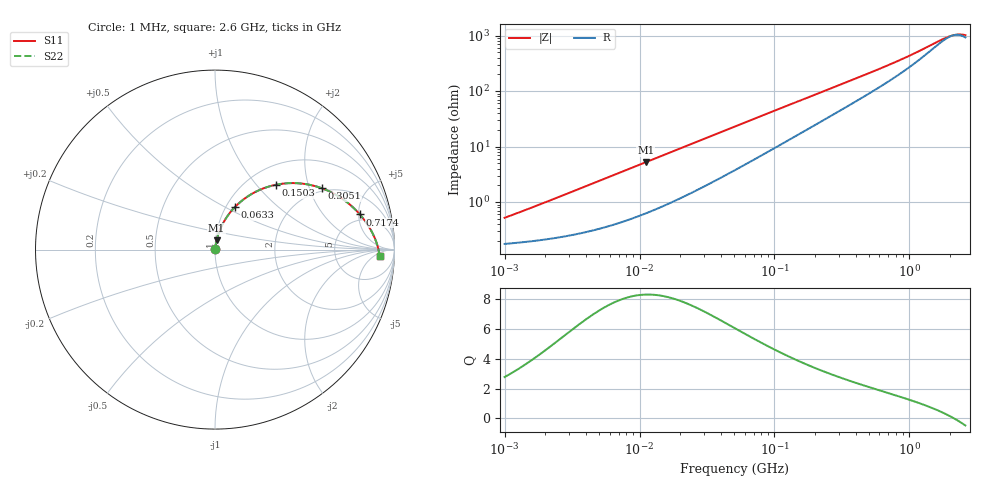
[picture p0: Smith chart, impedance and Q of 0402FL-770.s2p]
# MHz S MA R 50
!Freq  MagS11  AngS11  MagS21  AngS21  MagS12  AngS12  MagS22  AngS22
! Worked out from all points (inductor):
!   801 points, 1 MHz to 2.6 GHz, reference 50 ohm
!   read as one part in series: L = 77.1 nH near 1.103 MHz
!   highest Q = 8.32 at 11.11 MHz (marker M1), where L = 74 nH
!   self-resonance near 2.15 GHz
!   S11 on the Smith chart (normalised r, x): 1 MHz: 1.00, +0.01; 63.3 MHz: 1.10, +0.56; 150.3 MHz: 1.33, +1.27; 305.1 MHz: 1.88, +2.43; 717.4 MHz: 4.10, +5.18; 2.6 GHz: 19, -9
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1  0.005169 69.9  0.9982 -0.3  0.9982 -0.3  0.005169 69.9
1.526001  0.007615 74.9  0.998 -0.4  0.998 -0.4  0.007615 74.9
3.732571  0.01791 80.2  0.9971 -1.0  0.9971 -1.0  0.01791 80.2
11.11311  0.05167 80.2  0.9925 -2.9  0.9925 -2.9  0.05167 80.2
13.79581  0.06369 79.5  0.9904 -3.6  0.9904 -3.6  0.06369 79.5
27.18246  0.1218 75.4  0.9763 -6.9  0.9763 -6.9  0.1218 75.4
37.96865  0.1662 72.1  0.9619 -9.5  0.9619 -9.5  0.1662 72.1
50.9902  0.2167 68.3  0.9416 -12.3  0.9416 -12.3  0.2167 68.3
63.29923  0.2613 64.9  0.9203 -14.9  0.9203 -14.9  0.2613 64.9
96.59469  0.3665 57.0  0.8572 -21.0  0.8572 -21.0  0.3665 57.0
150.3299  0.4942 46.9  0.7544 -28.6  0.7544 -28.6  0.4942 46.9
190.3245  0.563 41.2  0.685 -32.7  0.685 -32.7  0.563 41.2
238.6026  0.6253 35.7  0.6123 -36.5  0.6123 -36.5  0.6253 35.7
305.0655  0.6861 29.9  0.5303 -40.2  0.5303 -40.2  0.6861 29.9
460.977  0.7683 21.2  0.3976 -44.4  0.3976 -44.4  0.7683 21.2
703.4513  0.8282 14.0  0.2801 -45.5  0.2801 -45.5  0.8282 14.0
717.4167  0.8305 13.7  0.2752 -45.5  0.2752 -45.5  0.8305 13.7
1052.571  0.8679 8.3  0.189 -41.6  0.189 -41.6  0.8679 8.3
1703.8  0.9 2.6  0.109 -22.2  0.109 -22.2  0.9 2.6
1936.029  0.9064 1.2  0.09567 -11.3  0.09567 -11.3  0.9064 1.2
2243.585  0.9126 -0.5  0.08776 5.0  0.08776 5.0  0.9126 -0.5
2600  0.9177 -2.2  0.09003 22.8  0.09003 22.8  0.9177 -2.2
